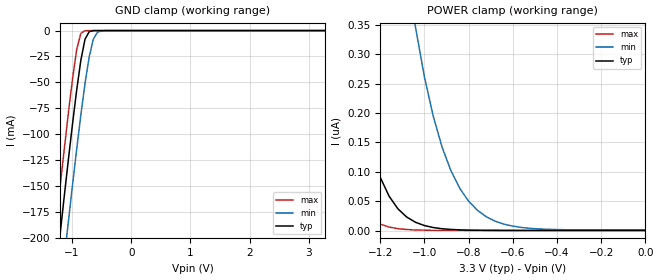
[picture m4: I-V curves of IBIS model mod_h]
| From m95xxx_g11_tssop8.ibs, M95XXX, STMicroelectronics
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|   Model mod_h
[Model]   mod_h
Model_type Input
Vinl   =   1.000V
Vinh   =   2.300V
C_comp   2.119pF   2.024pF   2.323pF
[Temperature Range]  25.0000   0.1050k   -40.0000
[Voltage Range]   3.3000V   2.7000V   3.6000V
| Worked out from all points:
|   GND clamp passes 1 mA (typ) near -0.70 V on its own axis
[GND_clamp]
|Voltage   I(typ)   I(min)   I(max)
-3.3V     -1.355A    -1.412A    -1.313A
-1.34V    -270.3mA   -330.7mA   -224.8mA
-1.27V    -233mA     -293.4mA   -187.4mA
-1.2V     -196.1mA   -256.5mA   -150.5mA
-1.13V    -159.7mA   -219.9mA   -114.2mA
-1.06V    -124.1mA   -183.9mA   -79.16mA
-920mV    -57.12mA   -114.2mA   -18.15mA
-850mV    -28.51mA   -81.35mA   -2.609mA
-780mV    -8.357mA   -51.08mA   -131.1uA
-640mV    -95.71uA   -8.329mA   -224.5nA
-500mV    -655.8nA   -243.4uA   -381.5pA
3.28V     6.871pA    315.5pA    6.69pA
[POWER_clamp]
|Voltage   I(typ)   I(min)   I(max)
-3.28V    7.333uA    8.217uA    7.391uA
-1.48V    902.4nA    1.702uA    394.5nA
-1.36V    399.2nA    1.511uA    106.3nA
-1.32V    288.1nA    1.424uA    63.11nA
-1.28V    201.9nA    1.253uA    36.16nA
-1.2V     90.95nA    871.6nA    10.96nA
-1.04V    13.98nA    345.9nA    900.7pA
-920mV    3.018nA    142.1nA    175.6pA
-840mV    1.082nA    71.85nA    89.07pA
-760mV    405.8pA    34.38nA    66.77pA
-560mV    74.59pA    5.144nA    59.57pA
0V        47.31pA    772.7pA    51.35pA
